FUNCTION_BLOCK "SIKO_DRV_POS_AG04B"
TITLE =
//KNOW_HOW_PROTECT
VERSION : 0.1


VAR_INPUT
  STARTADDRESS_STW : WORD ;	//PERIPHERY_STARTADDRESS_CONTROLBLOCK [HEX ]
  STARTADDRESS_ZSW : WORD ;	//PERIPHERY_STARTADDRESS_STATUSBLOCK [HEX ]
  POS_TARGET_VALUE : DINT ;	//Position Target Value -9999999 to 9999999
  OFF1 : BOOL ;	//STW Bit0 1=TRUE: Operating Condition
  OFF2 : BOOL ;	//STW Bit1 1=TRUE: Operating Condition
  OFF3 : BOOL ;	//STW Bit2  (not implemented)
  OPERATION_ENABLE : BOOL ;	//STW Bit3 1=TRUE: Operation Enable Operating Condition
  STOP : BOOL ;	//STW Bit4 1=TRUE: Operating Condition Positioning
  INTERMEDIATE_STOP : BOOL ;	//STW Bit5 1=TRUE: Operating Condition, 0=Positining interrupted
  AKTIVATE_TRAVEL_JOB : BOOL ;	//STW Bit6 Egde Enables New Travelling Job
  ACKNOWLEDGEMENT : BOOL ;	//STW Bit7 1=TRUE: Acklowledge Fault
  INCHING_1 : BOOL ;	//STW Bit8 1=TRUE: Drives Travels Once by Delta-Inch Target Value
  INCHING_2 : BOOL ;	//STW Bit9 1=TRUE: Drives Travels by a-Inch. Dircetion by Bit 15
  Bit10 : BOOL ;	//STW Bit10 Not Supported
  Bit11 : BOOL ;	//STW Bit11 Not Supported
  Bit12 : BOOL ;	//STW Bit12 Not Supported
  Bit13 : BOOL ;	//STW Bit13 Not Supported
  Bit14 : BOOL ;	//STW Bit14 Not Supported
  NEG_INCHING_2 : BOOL ;	//STW Bit15 1=TRUE: Negative Inching 2 Direction
  START_READ : BOOL ;
  START_WRITE : BOOL ;
  ENABLE_CALIBRATION : BOOL ;
END_VAR
VAR_OUTPUT
  POSITION_ACTUAL_VALUE : DINT ;	//Position Actual Value -9999999 to 9999999
  READY_TO_TURN_ON : BOOL ;	//ZSW Bit0 Supply voltage for motor and electronics unit applied
  READY_TO_TURN : BOOL ;	//ZSW Bit1 Supply voltage for motor and electronics unit applied
  OPERATION_ENABLED : BOOL ;	//ZSW Bit2 1=Positioning operation enabled
  ERROR : BOOL ;	//ZSW Bit3 1=Drive faulty and, therefore, out of operation
  NO_OFF_2 : BOOL ;	//ZSW Bit4 1=No pending OFF 2 command
  NO_OFF_3 : BOOL ;	//ZSW Bit5 Not implemented (statically on '1')
  TURN_ON_DISABLED : BOOL ;	//ZSW Bit6 1=Restart only via “OFF 1” with subsequent “On”
  WARNING : BOOL ;	//ZSW Bit7 1=Drive still in operation, no acknowledgement required
  NO_LAG_ERROR : BOOL ;	//ZSW Bit8 1=No lag error present
  GUIDE_REQUIRED : BOOL ;	//ZSW Bit9 Not supported (statically on ‘1’)
  TARGET_POSITION_REACHED : BOOL ;	//ZSW Bit10 1=Position value is at the end of a travel job in  positioning window
  REFERENCE_POINT_SET : BOOL ;	//ZSW Bit11 Not implemented - absolute system (statically on ‘1’).
  ACK_TARGET_VALUE : BOOL ;	//ZSW Bit12 ‘Edge’ acknowledges that a new positioning job was taken over
  DRIVE_STAND_STILL : BOOL ;	//ZSW Bit13 1=Signals standstill in case of intermediate stop and stop
  LIMIT_VALUE_EXCEEDED : BOOL ;	//ZSW Bit14 1=Position limiting value exceeded in pos. or neg. direction.
  READY_TO_TRAVEL : BOOL ;	//ZSW Bit15 1=AG is ready-to-travel if operation has been enabled
  DI_ES1 : BOOL ;	//Digital Input ES1 at AG04B
  DI_ES2 : BOOL ;	//Digital Input ES1 at AG04B
  DI_DI1 : BOOL ;	//Digital Input ES1 at AG04B
  DI_DI2 : BOOL ;	//Digital Input ES1 at AG04B
  DO_DI_ENABLE : BOOL ;	//Status of Enable at AG04B
  DO_MO_TORQUEDEACTIVATION : BOOL ;	//Status of Torque deactivation at AG04B
  COUNT_READ : INT ;
  COUNT_WRITE : INT ;
  Fault_SFC14 : INT ;
  Fault_SFC15 : INT ;
END_VAR
VAR
  Profibus_Address_r : WORD ;	//Address: 918 dez/ 396 hex Profibus Address r
  Operation_Mode_r : WORD  := W#16#2;	//Address: 930 dez/ 3A2 hex Operation Mode r/w
  Operation_Mode_w : WORD  := W#16#2;	//Address: 930 dez/ 3A2 hex Operation Mode r/w
  Fault_Buffer_r : ARRAY  [0 .. 9 ] OF WORD ;
  Number_of_Faults_r : WORD ;	//Address: 952 dez/ 3B8 hex Number of Faults r
  Hardware_Version_r : WORD ;	//Address: 961 dez/ 3C1 hex Hardware Version r
  Software_Version_r : WORD ;	//Address: 965 dez/ 3C5 hex Software Version r
  Parameter_Transfer_w : WORD ;	//Address: 970 dez/ 3CA hex Parameter Transfer w
  Controller_Parameter_P_r : WORD  := W#16#64;	//Address: 1000 dez/ 3E8 hex Controller Parameter P r/w
  Controller_Parameter_P_w : WORD  := W#16#64;	//Address: 1000 dez/ 3E8 hex Controller Parameter P r/w
  Controller_Parameter_I_r : WORD  := W#16#5;	//Address: 1001 dez/ 3E9 hex Controller Parameter I r/w
  Controller_Parameter_I_w : WORD  := W#16#5;	//Address: 1001 dez/ 3E9 hex Controller Parameter I r/w
  Controller_Parameter_D_r : WORD ;	//Address: 1002 dez/ 3EA hex Controller Parameter D r/w
  Controller_Parameter_D_w : WORD ;	//Address: 1002 dez/ 3EA hex Controller Parameter D r/w
  a_Pos_r : WORD  := W#16#32;	//Address: 1003 dez/ 3EB hex a_Pos r/w
  a_Pos_w : WORD  := W#16#32;	//Address: 1003 dez/ 3EB hex a_Pos r/w
  v_Pos_r : WORD  := W#16#1E;	//Address: 1004 dez/ 3EC hex v_Pos r/w
  v_Pos_w : WORD  := W#16#1E;	//Address: 1004 dez/ 3EC hex v_Pos r/w
  a_Rot_r : WORD  := W#16#32;	//Address: 1005 dez/ 3ED hex a_Rot r/w
  a_Rot_w : WORD  := W#16#32;	//Address: 1005 dez/ 3ED hex a_Rot r/w
  reserved_1_r : WORD ;	//Address: 1006 dez/ 3EE hex reserved 1 r/w
  reserved_1_w : WORD ;	//Address: 1006 dez/ 3EE hex reserved 1 r/w
  a_Inch_r : WORD  := W#16#32;	//Address: 1007 dez/ 3EF hex a_Inch r/w
  a_Inch_w : WORD  := W#16#32;	//Address: 1007 dez/ 3EF hex a_Inch r/w
  v_Inch_r : WORD  := W#16#1E;	//Address: 1008 dez/ 3F0 hex v_Inch r/w
  v_Inch_w : WORD  := W#16#1E;	//Address: 1008 dez/ 3F0 hex v_Inch r/w
  Pos_Window_r : WORD  := W#16#A;	//Address: 1009 dez/ 3F1 hex Pos Window r/w
  Pos_Window_w : WORD  := W#16#A;	//Address: 1009 dez/ 3F1 hex Pos Window r/w
  ue_Numerator_r : WORD  := W#16#1;	//Address: 1010 dez/ 3F2 hex ue_Numerator r/w
  ue_Numerator_w : WORD  := W#16#1;	//Address: 1010 dez/ 3F2 hex ue_Numerator r/w
  ue_Denominator_r : WORD  := W#16#1;	//Address: 1011 dez/ 3F3 hex ue_Denominator r/w
  ue_Denominator_w : WORD  := W#16#1;	//Address: 1011 dez/ 3F3 hex ue_Denominator r/w
  Spindle_Pitch_r : WORD ;	//Address: 1012 dez/ 3F4 hex Spindle Pitch r/w
  Spindle_Pitch_w : WORD ;	//Address: 1012 dez/ 3F4 hex Spindle Pitch r/w
  Sence_of_Rotation_r : WORD ;	//Address: 1013 dez/ 3F5 hex Sence of Rotation r/w
  Sence_of_Rotation_w : WORD ;	//Address: 1013 dez/ 3F5 hex Sence of Rotation r/w
  Pos_Type_r : WORD ;	//Address: 1014 dez/ 3F6 hex Pos Type r/w
  Pos_Type_w : WORD ;	//Address: 1014 dez/ 3F6 hex Pos Type r/w
  reserved_2_r : WORD ;	//Address: 1015 dez/ 3F7 hex resereserved 2
  reserved_2_w : WORD ;	//Address: 1015 dez/ 3F7 hex resereserved 2
  Upper_Limit_r : DWORD  := DW#16#186A0;	//Address: 1016 dez/ 3F8 hex Upper Limit r/w
  Upper_Limit_w : DWORD  := DW#16#186A0;	//Address: 1016 dez/ 3F8 hex Upper Limit r/w
  Lower_Limit_r : DWORD  := DW#16#FFFE7960;	//Address: 1017 dez/ 3F9 hex Lower Limit r/w
  Lower_Limit_w : DWORD  := DW#16#FFFE7960;	//Address: 1017 dez/ 3F9 hex Lower Limit r/w
  Calibration_Value_r : DWORD ;	//Address: 1018 dez/ 3FA hex Calibration Value r/w
  Calibration_Value_w : DWORD ;	//Address: 1018 dez/ 3FA hex Calibration Value r/w
  Delta_Inch_r : DWORD  := DW#16#400;	//Address: 1019 dez/ 3FB hex Delta Inch r/w
  Delta_Inch_w : DWORD  := DW#16#400;	//Address: 1019 dez/ 3FB hex Delta Inch r/w
  System_Status_Word_r : WORD ;	//Address: 1020 dez/ 3FC hex System Status Word r
  StoppMode_Inch2_r : WORD ;	//Address: 1021 dez/ 3FD hex Stopp-Mode Inch2 r/w
  StoppMode_Inch2_w : WORD ;	//Address: 1021 dez/ 3FD hex Stopp-Mode Inch2 r/w
  InPos_Mode_r : WORD ;	//Adresse: 1022 dez/ 3FE hex InPos_Mode r/w
  InPos_Mode_w : WORD ;	//Adresse: 1022 dez/ 3FE hex InPos_Mode r/w
  Loop_length_r : WORD  := W#16#200;	//Adresse: 1023 dez/ 3FF hex Loop_length r/w
  Loop_length_w : WORD  := W#16#200;	//Adresse: 1023 dez/ 3FF hex Loop_length r/w
  Contouring_error_limit_r : WORD  := W#16#190;	//Adresse: 1024 dez/ 400 hex Loop_length r/w
  Contouring_error_limit_w : WORD  := W#16#190;	//Adresse: 1024 dez/ 400 hex Loop_length r/w
  Contouring_error_r : DWORD ;	//Adresse: 1025 dez/ 401 hex Contouring_error r
  Supply_voltage_r : WORD ;	//Adresse: 1026 dez/ 402 hex Supply_voltage r
  Device_temperature_r : WORD ;	//Adresse: 1027 dez/ 403 hex Device_temperature r
  Device_temperature_max_r : WORD ;	//Adresse: 1028 dez/ 404 hex Device_temperature_max r
  Motor_current_r : WORD ;	//Adresse: 1029 dez/ 405 hex Motor_current r
  Motor_current_max_r : WORD ;	//Adresse: 1030 dez/ 406 hex Motor_current_max r
  Gen_Status_Register_r : WORD ;	//Adresse: 1031 dez/ 407 hex Digital_inputs r
  Torque_Deactivation_r : WORD  := W#16#7D;	//Adresse: 1032 dez/ 408 hex InPos_Mode r/w
  Torque_Deactivation_w : WORD  := W#16#7D;	//Adresse: 1032 dez/ 408 hex InPos_Mode r/w
  Serial_number_r : DWORD ;	//Adresse: 1033 dez/ 409 hex Serial_number r
  AF_OSR_START_WRITE : BOOL ;
  OSR_START_WRITE : BOOL ;
  AF_OSR_START_READ : BOOL ;
  OSR_START_READ : BOOL ;
  REFRESH : BOOL ;
  COUNTER_READ : INT ;
  COUNTER_WRITE : INT ;
END_VAR
VAR_TEMP
  DC_STEUERBEREICH_TEMP : ARRAY  [1 .. 14 ] OF //PERIEPHERIE_STEUERBEREICH_TEMP
  BYTE ;
  DC_ZUSTANDSBEREICH_TEMP : ARRAY  [1 .. 14 ] OF //PERIEPHERIE_ZUSTANDSBEREICH_TEMP
  BYTE ;
  Failure : INT ;
END_VAR
BEGIN
NETWORK
TITLE =STW 1
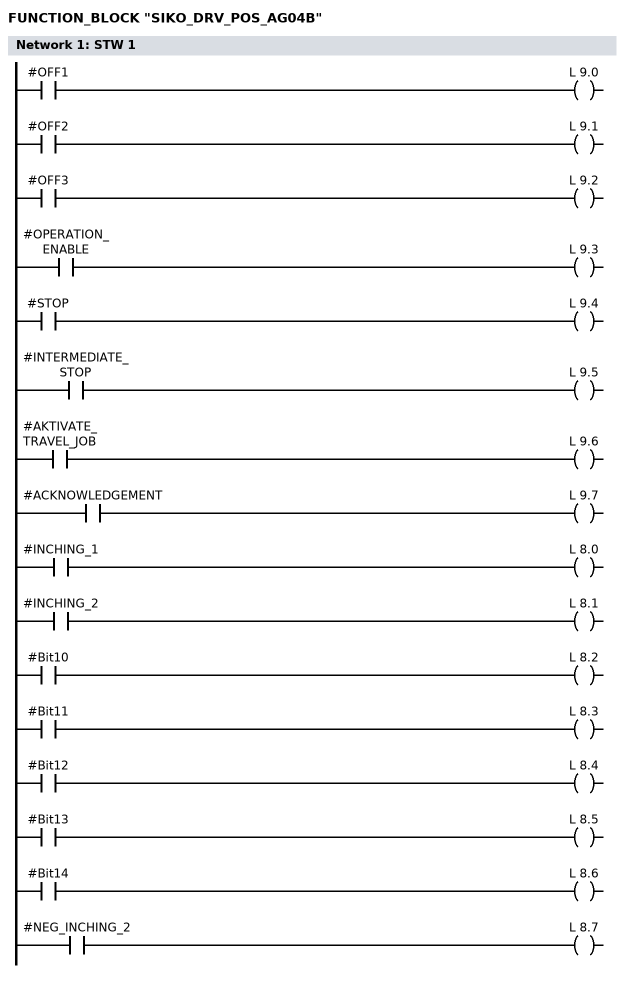
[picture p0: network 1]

      U     #OFF1;
      =     L      9.0;
      U     #OFF2;
      =     L      9.1;
      U     #OFF3;
      =     L      9.2;
      U     #OPERATION_ENABLE;
      =     L      9.3;
      U     #STOP;
      =     L      9.4;
      U     #INTERMEDIATE_STOP;
      =     L      9.5;
      U     #AKTIVATE_TRAVEL_JOB;
      =     L      9.6;
      U     #ACKNOWLEDGEMENT;
      =     L      9.7;
      U     #INCHING_1;
      =     L      8.0;
      U     #INCHING_2;
      =     L      8.1;
      U     #Bit10;
      =     L      8.2;
      U     #Bit11;
      =     L      8.3;
      U     #Bit12;
      =     L      8.4;
      U     #Bit13;
      =     L      8.5;
      U     #Bit14;
      =     L      8.6;
      U     #NEG_INCHING_2;
      =     L      8.7;

NETWORK
TITLE =CREATION OF SET POINT WORD (HSW/PZD2)
//PZD2
      L     #POS_TARGET_VALUE;
      L     L#-9999999;
      >D    ;
      SPB   M001;
      L     0;
      SPA   END0;
M001: L     #POS_TARGET_VALUE;
      L     L#9999999;
      <=D   ;
      SPB   M002;
      L     0;
      SPA   END0;
M002: L     #POS_TARGET_VALUE;
END0: T     LD    10;

NETWORK
TITLE =Start Read / Write Flanke
//Flanke bilden start lesen
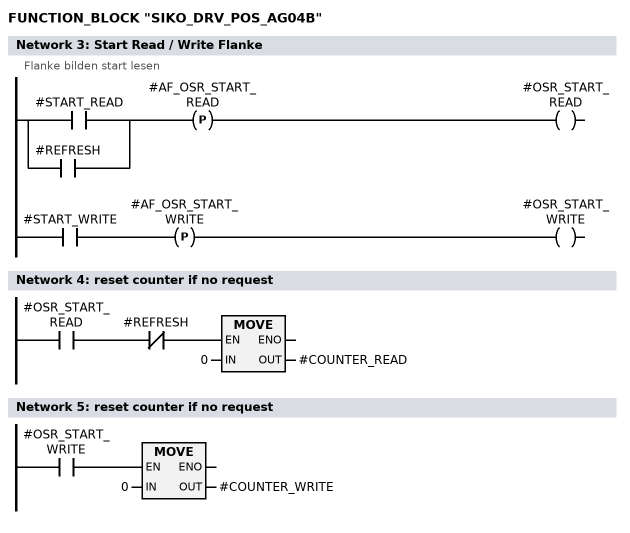
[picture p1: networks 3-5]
      O     #START_READ;
      O     #REFRESH;
      FP    #AF_OSR_START_READ;
      =     #OSR_START_READ;

//Flanke bilden start lesen
      U     #START_WRITE;
      FP    #AF_OSR_START_WRITE;
      =     #OSR_START_WRITE;



NETWORK
TITLE =reset counter if no request

      U     #OSR_START_READ;
      UN    #REFRESH;
      SPBNB _001;
      L     0;
      T     #COUNTER_READ;
_001: NOP   0;
NETWORK
TITLE =reset counter if no request

      U     #OSR_START_WRITE;
      SPBNB _002;
      L     0;
      T     #COUNTER_WRITE;
_002: NOP   0;
NETWORK
TITLE =Par Request read to drv
//
//
//Counter auf 1 bei start
      L     0;
      T     LW     0;
      U     #OSR_START_READ;
      SPBN  pa31;
      L     1;
      T     #COUNTER_READ;



//Parameter anfordern ************************************


//Profibus
pa31: L     #COUNTER_READ;
      L     1;
      ==I   ;
      SPBN  pa32;
      L     W#16#1396;
      T     LW     0;

//Betriebsart
pa32: L     #COUNTER_READ;
      L     2;
      ==I   ;
      SPBN  pa33;
      L     W#16#13A2;
      T     LW     0;

//Störspeicher 0
pa33: L     #COUNTER_READ;
      L     3;
      ==I   ;
      SPBN  pa34;
      L     W#16#63B1;
      T     LW     0;
      L     0;
      T     LW     2;
//Störspeicher 1
pa34: L     #COUNTER_READ;
      L     4;
      ==I   ;
      SPBN  pa35;
      L     W#16#63B1;
      T     LW     0;
      L     1;
      T     LW     2;
//Störspeicher 2
pa35: L     #COUNTER_READ;
      L     5;
      ==I   ;
      SPBN  pa36;
      L     W#16#63B1;
      T     LW     0;
      L     2;
      T     LW     2;
//Störspeicher 3
pa36: L     #COUNTER_READ;
      L     6;
      ==I   ;
      SPBN  pa37;
      L     W#16#63B1;
      T     LW     0;
      L     3;
      T     LW     2;
//Störspeicher 4
pa37: L     #COUNTER_READ;
      L     7;
      ==I   ;
      SPBN  pa38;
      L     W#16#63B1;
      T     LW     0;
      L     4;
      T     LW     2;
//Störspeicher 5
pa38: L     #COUNTER_READ;
      L     8;
      ==I   ;
      SPBN  pa39;
      L     W#16#63B1;
      T     LW     0;
      L     5;
      T     LW     2;
//Störspeicher 6
pa39: L     #COUNTER_READ;
      L     9;
      ==I   ;
      SPBN  pa40;
      L     W#16#63B1;
      T     LW     0;
      L     6;
      T     LW     2;
//Störspeicher 7
pa40: L     #COUNTER_READ;
      L     10;
      ==I   ;
      SPBN  pa41;
      L     W#16#63B1;
      T     LW     0;
      L     7;
      T     LW     2;
//Störspeicher 8
pa41: L     #COUNTER_READ;
      L     11;
      ==I   ;
      SPBN  pa42;
      L     W#16#63B1;
      T     LW     0;
      L     8;
      T     LW     2;
//Störspeicher 9
pa42: L     #COUNTER_READ;
      L     12;
      ==I   ;
      SPBN  pa43;
      L     W#16#63B1;
      T     LW     0;
      L     9;
      T     LW     2;

//Anzahl Störungen
pa43: L     #COUNTER_READ;
      L     13;
      ==I   ;
      SPBN  pa44;
      L     W#16#13B8;
      T     LW     0;

//Hardware-Version
pa44: L     #COUNTER_READ;
      L     14;
      ==I   ;
      SPBN  pa45;
      L     W#16#13C1;
      T     LW     0;

//Software-Version
pa45: L     #COUNTER_READ;
      L     15;
      ==I   ;
      SPBN  pa46;
      L     W#16#13C5;
      T     LW     0;

//Regler-Parameter P-Anteil
pa46: L     #COUNTER_READ;
      L     16;
      ==I   ;
      SPBN  pa47;
      L     W#16#13E8;
      T     LW     0;

//Regler-Parameter I-Anteil
pa47: L     #COUNTER_READ;
      L     17;
      ==I   ;
      SPBN  pa48;
      L     W#16#13E9;
      T     LW     0;

//Regler-Parameter D-Anteil
pa48: L     #COUNTER_READ;
      L     18;
      ==I   ;
      SPBN  pa49;
      L     W#16#13EA;
      T     LW     0;

//a - Pos
pa49: L     #COUNTER_READ;
      L     19;
      ==I   ;
      SPBN  pa50;
      L     W#16#13EB;
      T     LW     0;

//v - Pos
pa50: L     #COUNTER_READ;
      L     20;
      ==I   ;
      SPBN  pa51;
      L     W#16#13EC;
      T     LW     0;

//a - Dreh
pa51: L     #COUNTER_READ;
      L     21;
      ==I   ;
      SPBN  pa52;
      L     W#16#13ED;
      T     LW     0;

//a - Tipp
pa52: L     #COUNTER_READ;
      L     22;
      ==I   ;
      SPBN  pa53;
      L     W#16#13EF;
      T     LW     0;

//v - Tipp
pa53: L     #COUNTER_READ;
      L     23;
      ==I   ;
      SPBN  pa54;
      L     W#16#13F0;
      T     LW     0;

//Pos - Fenster
pa54: L     #COUNTER_READ;
      L     24;
      ==I   ;
      SPBN  pa55;
      L     W#16#13F1;
      T     LW     0;

//ü - Zähler
pa55: L     #COUNTER_READ;
      L     25;
      ==I   ;
      SPBN  pa56;
      L     W#16#13F2;
      T     LW     0;

//ü - Nenner
pa56: L     #COUNTER_READ;
      L     26;
      ==I   ;
      SPBN  pa57;
      L     W#16#13F3;
      T     LW     0;

//Spindelsteigung
pa57: L     #COUNTER_READ;
      L     27;
      ==I   ;
      SPBN  pa58;
      L     W#16#13F4;
      T     LW     0;

//Drehrichtung
pa58: L     #COUNTER_READ;
      L     28;
      ==I   ;
      SPBN  pa59;
      L     W#16#13F5;
      T     LW     0;

//Pos-Art
pa59: L     #COUNTER_READ;
      L     29;
      ==I   ;
      SPBN  pa60;
      L     W#16#13F6;
      T     LW     0;

//Oberer Grenzwert
pa60: L     #COUNTER_READ;
      L     30;
      ==I   ;
      SPBN  pa61;
      L     W#16#13F8;
      T     LW     0;

//Unterer Grenzwert
pa61: L     #COUNTER_READ;
      L     31;
      ==I   ;
      SPBN  pa62;
      L     W#16#13F9;
      T     LW     0;

//Kalibrierwert
pa62: L     #COUNTER_READ;
      L     32;
      ==I   ;
      SPBN  pa63;
      L     W#16#13FA;
      T     LW     0;

//Delta Tipp
pa63: L     #COUNTER_READ;
      L     33;
      ==I   ;
      SPBN  pa64;
      L     W#16#13FB;
      T     LW     0;

//SYSTEM Statuswort
pa64: L     #COUNTER_READ;
      L     34;
      ==I   ;
      SPBN  pa65;
      L     W#16#13FC;
      T     LW     0;

//Stopp-Mode Tipp2
pa65: L     #COUNTER_READ;
      L     35;
      ==I   ;
      SPBN  pa66;
      L     W#16#13FD;
      T     LW     0;

//InPos-Mode
pa66: L     #COUNTER_READ;
      L     36;
      ==I   ;
      SPBN  pa67;
      L     W#16#13FE;
      T     LW     0;

//Schleifenlaenge
pa67: L     #COUNTER_READ;
      L     37;
      ==I   ;
      SPBN  pa68;
      L     W#16#13FF;
      T     LW     0;

//Schleppfehler_Grenze
pa68: L     #COUNTER_READ;
      L     38;
      ==I   ;
      SPBN  pa69;
      L     W#16#1400;
      T     LW     0;

//Schleppfehler
pa69: L     #COUNTER_READ;
      L     39;
      ==I   ;
      SPBN  pa70;
      L     W#16#1401;
      T     LW     0;

//Versorgungsspannung
pa70: L     #COUNTER_READ;
      L     40;
      ==I   ;
      SPBN  pa71;
      L     W#16#1402;
      T     LW     0;

//Geraetetemperatur
pa71: L     #COUNTER_READ;
      L     41;
      ==I   ;
      SPBN  pa72;
      L     W#16#1403;
      T     LW     0;

//Geraetetemperatur_Max
pa72: L     #COUNTER_READ;
      L     42;
      ==I   ;
      SPBN  pa73;
      L     W#16#1404;
      T     LW     0;

//Motorstrom
pa73: L     #COUNTER_READ;
      L     43;
      ==I   ;
      SPBN  pa74;
      L     W#16#1405;
      T     LW     0;

//Motorstrom_Max
pa74: L     #COUNTER_READ;
      L     44;
      ==I   ;
      SPBN  pa75;
      L     W#16#1406;
      T     LW     0;

//Digital_Eingaenge
pa75: L     #COUNTER_READ;
      L     45;
      ==I   ;
      SPBN  pa76;
      L     W#16#1407;
      T     LW     0;

//Drehmoment_Abschaltung
pa76: L     #COUNTER_READ;
      L     46;
      ==I   ;
      SPBN  pa77;
      L     W#16#1408;
      T     LW     0;

//Seriennummer
pa77: L     #COUNTER_READ;
      L     47;
      ==I   ;
      SPBN  pa99;
      L     W#16#1409;
      T     LW     0;

pa99: NOP   0; //ENDE


NETWORK
TITLE =Par Request write to drv
//
//
//
//
//Counter auf 1 bei start
      U     #OSR_START_WRITE;
      SPBN  pr61;
      L     1;
      T     #COUNTER_WRITE;


//Parameter anfordern ************************************
//Betriebsart
pr61: L     #COUNTER_WRITE;
      L     1;
      ==I   ;
      SPBN  pr62;
      L     #Operation_Mode_w;
      L     #Operation_Mode_r;
      ==I   ;
      SPB   co80;
      L     W#16#23A2;
      T     LW     0;
      L     #Operation_Mode_w;
      T     LD     4;

//Reglerparameter_P
pr62: L     #COUNTER_WRITE;
      L     2;
      ==I   ;
      SPBN  pr63;
      L     #Controller_Parameter_P_w;
      L     #Controller_Parameter_P_r;
      ==I   ;
      SPB   co80;
      L     W#16#23E8;
      T     LW     0;
      L     #Controller_Parameter_P_w;
      T     LD     4;

//Reglerparameter_I
pr63: L     #COUNTER_WRITE;
      L     3;
      ==I   ;
      SPBN  pr64;
      L     #Controller_Parameter_I_w;
      L     #Controller_Parameter_I_r;
      ==I   ;
      SPB   co80;
      L     W#16#23E9;
      T     LW     0;
      L     #Controller_Parameter_I_w;
      T     LD     4;

//Reglerparameter_D
pr64: L     #COUNTER_WRITE;
      L     4;
      ==I   ;
      SPBN  pr65;
      L     #Controller_Parameter_D_w;
      L     #Controller_Parameter_D_r;
      ==I   ;
      SPB   co80;
      L     W#16#23EA;
      T     LW     0;
      L     #Controller_Parameter_D_w;
      T     LD     4;

//a_Pos
pr65: L     #COUNTER_WRITE;
      L     5;
      ==I   ;
      SPBN  pr66;
      L     #a_Pos_w;
      L     #a_Pos_r;
      ==I   ;
      SPB   co80;
      L     W#16#23EB;
      T     LW     0;
      L     #a_Pos_w;
      T     LD     4;

//v_Pos
pr66: L     #COUNTER_WRITE;
      L     6;
      ==I   ;
      SPBN  pr67;
      L     #v_Pos_w;
      L     #v_Pos_r;
      ==I   ;
      SPB   co80;
      L     W#16#23EC;
      T     LW     0;
      L     #v_Pos_w;
      T     LD     4;

//a_Dreh
pr67: L     #COUNTER_WRITE;
      L     7;
      ==I   ;
      SPBN  pr68;
      L     #a_Rot_w;
      L     #a_Rot_r;
      ==I   ;
      SPB   co80;
      L     W#16#23ED;
      T     LW     0;
      L     #a_Rot_w;
      T     LD     4;

//a_Tipp
pr68: L     #COUNTER_WRITE;
      L     8;
      ==I   ;
      SPBN  pr69;
      L     #a_Inch_w;
      L     #a_Inch_r;
      ==I   ;
      SPB   co80;
      L     W#16#23EF;
      T     LW     0;
      L     #a_Inch_w;
      T     LD     4;

//v_Tip
pr69: L     #COUNTER_WRITE;
      L     9;
      ==I   ;
      SPBN  pr70;
      L     #v_Inch_w;
      L     #v_Inch_r;
      ==I   ;
      SPB   co80;
      L     W#16#23F0;
      T     LW     0;
      L     #v_Inch_w;
      T     LD     4;

//Pos_Fenster
pr70: L     #COUNTER_WRITE;
      L     10;
      ==I   ;
      SPBN  pr71;
      L     #Pos_Window_w;
      L     #Pos_Window_r;
      ==I   ;
      SPB   co80;
      L     W#16#23F1;
      T     LW     0;
      L     #Pos_Window_w;
      T     LD     4;

//ue_Zaehler
pr71: L     #COUNTER_WRITE;
      L     11;
      ==I   ;
      SPBN  pr72;
      L     #ue_Numerator_w;
      L     #ue_Numerator_r;
      ==I   ;
      SPB   co80;
      L     W#16#23F2;
      T     LW     0;
      L     #ue_Numerator_w;
      T     LD     4;

//ue_Nenner
pr72: L     #COUNTER_WRITE;
      L     12;
      ==I   ;
      SPBN  pr73;
      L     #ue_Denominator_w;
      L     #ue_Denominator_r;
      ==I   ;
      SPB   co80;
      L     W#16#23F3;
      T     LW     0;
      L     #ue_Denominator_w;
      T     LD     4;

//Spindelsteigung
pr73: L     #COUNTER_WRITE;
      L     13;
      ==I   ;
      SPBN  pr74;
      L     #Spindle_Pitch_w;
      L     #Spindle_Pitch_r;
      ==I   ;
      SPB   co80;
      L     W#16#23F4;
      T     LW     0;
      L     #Spindle_Pitch_w;
      T     LD     4;

//Drehrichtung
pr74: L     #COUNTER_WRITE;
      L     14;
      ==I   ;
      SPBN  pr75;
      L     #Sence_of_Rotation_w;
      L     #Sence_of_Rotation_r;
      ==I   ;
      SPB   co80;
      L     W#16#23F5;
      T     LW     0;
      L     #Sence_of_Rotation_w;
      T     LD     4;

//Pos_Art_
pr75: L     #COUNTER_WRITE;
      L     15;
      ==I   ;
      SPBN  pr76;
      L     #Pos_Type_w;
      L     #Pos_Type_r;
      ==I   ;
      SPB   co80;
      L     W#16#23F6;
      T     LW     0;
      L     #Pos_Type_w;
      T     LD     4;

//oberer_Grenzwert
pr76: L     #COUNTER_WRITE;
      L     16;
      ==I   ;
      SPBN  pr77;
      L     #Upper_Limit_w;
      L     #Upper_Limit_r;
      ==I   ;
      SPB   co80;
      L     W#16#33F8;
      T     LW     0;
      L     #Upper_Limit_w;
      T     LD     4;

//unterer_Grenzwert
pr77: L     #COUNTER_WRITE;
      L     17;
      ==I   ;
      SPBN  pr78;
      L     #Lower_Limit_w;
      L     #Lower_Limit_r;
      ==I   ;
      SPB   co80;
      L     W#16#33F9;
      T     LW     0;
      L     #Lower_Limit_w;
      T     LD     4;

//Kalibrierwert
pr78: L     #COUNTER_WRITE;
      L     18;
      ==I   ;
      SPBN  pr79;
//L     #Calibration_Value_w
//L     #Calibration_Value_r
//==I
      UN    #ENABLE_CALIBRATION;
      SPB   co80;
      L     W#16#33FA;
      T     LW     0;
      L     #Calibration_Value_w;
      T     LD     4;

//Delta_Tipp
pr79: L     #COUNTER_WRITE;
      L     19;
      ==I   ;
      SPBN  pr80;
      L     #Delta_Inch_w;
      L     #Delta_Inch_r;
      ==I   ;
      SPB   co80;
      L     W#16#33FB;
      T     LW     0;
      L     #Delta_Inch_w;
      T     LD     4;

//Stopp-Mode Tipp2
pr80: L     #COUNTER_WRITE;
      L     20;
      ==I   ;
      SPBN  pr81;
      L     #StoppMode_Inch2_w;
      L     #StoppMode_Inch2_r;
      ==I   ;
      SPB   co80;
      L     W#16#23FD;
      T     LW     0;
      L     #StoppMode_Inch2_w;
      T     LD     4;

//InPos_Mode
pr81: L     #COUNTER_WRITE;
      L     21;
      ==I   ;
      SPBN  pl82;
      L     #InPos_Mode_w;
      L     #InPos_Mode_r;
      ==I   ;
      SPB   co80;
      L     W#16#23FE;
      T     LW     0;
      L     #InPos_Mode_w;
      T     LD     4;

//Schleifenlaenge
pl82: L     #COUNTER_WRITE;
      L     22;
      ==I   ;
      SPBN  pl83;
      L     #Loop_length_w;
      L     #Loop_length_r;
      ==I   ;
      SPB   co80;
      L     W#16#23FF;
      T     LW     0;
      L     #Loop_length_w;
      T     LD     4;

//Schleppfehler_Grenze
pl83: L     #COUNTER_WRITE;
      L     23;
      ==I   ;
      SPBN  pl84;
      L     #Contouring_error_limit_w;
      L     #Contouring_error_limit_r;
      ==I   ;
      SPB   co80;
      L     W#16#2400;
      T     LW     0;
      L     #Contouring_error_limit_w;
      T     LD     4;

//Drehmoment_Abschaltung
pl84: L     #COUNTER_WRITE;
      L     24;
      ==I   ;
      SPBN  pz99;
      L     #Torque_Deactivation_w;
      L     #Torque_Deactivation_r;
      ==I   ;
      SPB   co80;
      L     W#16#2408;
      T     LW     0;
      L     #Torque_Deactivation_w;
      T     LD     4;

//Parametersatz laden
pz99: L     #COUNTER_WRITE;
      L     25;
      ==I   ;
      SPBN  end6;
      L     W#16#23CA;
      T     LW     0;
      L     #Parameter_Transfer_w;
      T     LD     4;

      SPA   end6;


//erhöhe Zähler wenn kein schreiben notwendig
// Zähler +1
co80: L     #COUNTER_WRITE;
      INC   1;
      T     #COUNTER_WRITE;

end6: NOP   0; //ENDE



NETWORK
TITLE =
//Eingänge abfragen, wenn Parameterabgleich inaktiv
      L     0;
      L     #COUNT_WRITE;
      ==I   ;
      SPBN  xyy1;
      L     0;
      L     #COUNT_READ;
      ==I   ;
      SPBN  xyy1;
      L     W#16#1407;
      T     LW     0;

xyy1: NOP   0;


NETWORK
TITLE =transmit to drive

      CALL "DPWR_DAT" (
           LADDR                    := #STARTADDRESS_STW,
           RECORD                   := P#L 0.0 BYTE 14,
           RET_VAL                  := #Fault_SFC15);
      NOP   0;
NETWORK
TITLE =Read from Drive

      CALL "DPRD_DAT" (
           LADDR                    := #STARTADDRESS_ZSW,
           RET_VAL                  := #Fault_SFC14,
           RECORD                   := P#L 14.0 BYTE 14);
      NOP   0;

NETWORK
TITLE =
//Eingänge abfragen, wenn Parameterabgleich inaktiv
      L     0;
      L     #COUNT_WRITE;
      ==I   ;
      SPBN  xxy1;
      L     0;
      L     #COUNT_READ;
      ==I   ;
      SPBN  xxy1;
      L     LW    14;
      L     W#16#1407;
      ==I   ;
      SPBN  xxy1;

      U     L     21.0;
      =     #DI_ES1;
      U     L     21.1;
      =     #DI_ES2;
      U     L     21.2;
      =     #DI_DI1;
      U     L     21.3;
      =     #DI_DI2;
      U     L     21.4;
      =     #DO_DI_ENABLE;
      U     L     21.7;
      =     #DO_MO_TORQUEDEACTIVATION;

xxy1: NOP   0;


NETWORK
TITLE =read par from drv (read)
//
//
      L     #COUNTER_READ; //Zählerstand nach aussen geben
      T     #COUNT_READ; //Zählerstand nach aussen geben
//Profibus
      L     #COUNTER_READ; //Parameterwert auslesen START
      L     1;
      ==I   ;
      SPBN  rp2;
      L     LW    14;
      L     W#16#1396;
      ==I   ;
      SPBN  end9;
      L     LD    18;
      T     #Profibus_Address_r;
// Zähler +1
      L     #COUNTER_READ;
      INC   1;
      T     #COUNTER_READ; //Parameterwert auslesen ENDE

//Betriebsart
rp2:  L     #COUNTER_READ; //Parameterwert auslesen START
      L     2;
      ==I   ;
      SPBN  rp3;
      L     LW    14;
      L     W#16#13A2;
      ==I   ;
      SPBN  end9;
      L     LD    18;
      T     #Operation_Mode_r;
// Zähler +1
      L     #COUNTER_READ;
      INC   1;
      T     #COUNTER_READ; //Parameterwert auslesen ENDE

//Störspeicher 0
rp3:  L     #COUNTER_READ; //Parameterwert auslesen START
      L     3;
      ==I   ;
      SPBN  rp4;
      L     LW    14;
      L     W#16#43B1;
      ==I   ;
      SPBN  end9;
      L     LW    16;
      L     0;
      ==I   ;
      SPBN  end9;
      L     LD    18;
      T     #Fault_Buffer_r[0];
// Zähler +1
      L     #COUNTER_READ;
      INC   1;
      T     #COUNTER_READ; //Parameterwert auslesen ENDE

//Störspeicher 1
rp4:  L     #COUNTER_READ; //Parameterwert auslesen START
      L     4;
      ==I   ;
      SPBN  rp5;
      L     LW    14;
      L     W#16#43B1;
      ==I   ;
      SPBN  end9;
      L     LW    16;
      L     1;
      ==I   ;
      SPBN  end9;
      L     LD    18;
      T     #Fault_Buffer_r[1];
// Zähler +1
      L     #COUNTER_READ;
      INC   1;
      T     #COUNTER_READ; //Parameterwert auslesen ENDE

//Störspeicher 2
rp5:  L     #COUNTER_READ; //Parameterwert auslesen START
      L     5;
      ==I   ;
      SPBN  rp6;
      L     LW    14;
      L     W#16#43B1;
      ==I   ;
      SPBN  end9;
      L     LW    16;
      L     2;
      ==I   ;
      SPBN  end9;
      L     LD    18;
      T     #Fault_Buffer_r[2];
// Zähler +1
      L     #COUNTER_READ;
      INC   1;
      T     #COUNTER_READ; //Parameterwert auslesen ENDE

//Störspeicher 3
rp6:  L     #COUNTER_READ; //Parameterwert auslesen START
      L     6;
      ==I   ;
      SPBN  rp7;
      L     LW    14;
      L     W#16#43B1;
      ==I   ;
      SPBN  end9;
      L     LW    16;
      L     3;
      ==I   ;
      SPBN  end9;
      L     LD    18;
      T     #Fault_Buffer_r[3];
// Zähler +1
      L     #COUNTER_READ;
      INC   1;
      T     #COUNTER_READ; //Parameterwert auslesen ENDE

//Störspeicher 4
rp7:  L     #COUNTER_READ; //Parameterwert auslesen START
      L     7;
      ==I   ;
      SPBN  rp8;
      L     LW    14;
      L     W#16#43B1;
      ==I   ;
      SPBN  end9;
      L     LW    16;
      L     4;
      ==I   ;
      SPBN  end9;
      L     LD    18;
      T     #Fault_Buffer_r[4];
// Zähler +1
      L     #COUNTER_READ;
      INC   1;
      T     #COUNTER_READ; //Parameterwert auslesen ENDE

//Störspeicher 5
rp8:  L     #COUNTER_READ; //Parameterwert auslesen START
      L     8;
      ==I   ;
      SPBN  rp9;
      L     LW    14;
      L     W#16#43B1;
      ==I   ;
      SPBN  end9;
      L     LW    16;
      L     5;
      ==I   ;
      SPBN  end9;
      L     LD    18;
      T     #Fault_Buffer_r[5];
// Zähler +1
      L     #COUNTER_READ;
      INC   1;
      T     #COUNTER_READ; //Parameterwert auslesen ENDE

//Störspeicher 6
rp9:  L     #COUNTER_READ; //Parameterwert auslesen START
      L     9;
      ==I   ;
      SPBN  rp10;
      L     LW    14;
      L     W#16#43B1;
      ==I   ;
      SPBN  end9;
      L     LW    16;
      L     6;
      ==I   ;
      SPBN  end9;
      L     LD    18;
      T     #Fault_Buffer_r[6];
// Zähler +1
      L     #COUNTER_READ;
      INC   1;
      T     #COUNTER_READ; //Parameterwert auslesen ENDE

//Störspeicher 7
rp10: L     #COUNTER_READ; //Parameterwert auslesen START
      L     10;
      ==I   ;
      SPBN  rp11;
      L     LW    14;
      L     W#16#43B1;
      ==I   ;
      SPBN  end9;
      L     LW    16;
      L     7;
      ==I   ;
      SPBN  end9;
      L     LD    18;
      T     #Fault_Buffer_r[7];
// Zähler +1
      L     #COUNTER_READ;
      INC   1;
      T     #COUNTER_READ; //Parameterwert auslesen ENDE

//Störspeicher 8
rp11: L     #COUNTER_READ; //Parameterwert auslesen START
      L     11;
      ==I   ;
      SPBN  rp12;
      L     LW    14;
      L     W#16#43B1;
      ==I   ;
      SPBN  end9;
      L     LW    16;
      L     8;
      ==I   ;
      SPBN  end9;
      L     LD    18;
      T     #Fault_Buffer_r[8];
// Zähler +1
      L     #COUNTER_READ;
      INC   1;
      T     #COUNTER_READ; //Parameterwert auslesen ENDE

//Störspeicher 9
rp12: L     #COUNTER_READ; //Parameterwert auslesen START
      L     12;
      ==I   ;
      SPBN  rp13;
      L     LW    14;
      L     W#16#43B1;
      ==I   ;
      SPBN  end9;
      L     LW    16;
      L     9;
      ==I   ;
      SPBN  end9;
      L     LD    18;
      T     #Fault_Buffer_r[9];
// Zähler +1
      L     #COUNTER_READ;
      INC   1;
      T     #COUNTER_READ; //Parameterwert auslesen ENDE

//Anzahl Störungen
rp13: L     #COUNTER_READ; //Parameterwert auslesen START
      L     13;
      ==I   ;
      SPBN  rp14;
      L     LW    14;
      L     W#16#13B8;
      ==I   ;
      SPBN  end9;
      L     LD    18;
      T     #Number_of_Faults_r;
// Zähler +1
      L     #COUNTER_READ;
      INC   1;
      T     #COUNTER_READ; //Parameterwert auslesen ENDE

//Hardware-Version
rp14: L     #COUNTER_READ; //Parameterwert auslesen START
      L     14;
      ==I   ;
      SPBN  rp15;
      L     LW    14;
      L     W#16#13C1;
      ==I   ;
      SPBN  end9;
      L     LD    18;
      T     #Hardware_Version_r;
// Zähler +1
      L     #COUNTER_READ;
      INC   1;
      T     #COUNTER_READ; //Parameterwert auslesen ENDE

//Software-Version
rp15: L     #COUNTER_READ; //Parameterwert auslesen START
      L     15;
      ==I   ;
      SPBN  rp16;
      L     LW    14;
      L     W#16#13C5;
      ==I   ;
      SPBN  end9;
      L     LD    18;
      T     #Software_Version_r;
// Zähler +1
      L     #COUNTER_READ;
      INC   1;
      T     #COUNTER_READ; //Parameterwert auslesen ENDE

//Regler-Parameter P-Anteil
rp16: L     #COUNTER_READ; //Parameterwert auslesen START
      L     16;
      ==I   ;
      SPBN  rp17;
      L     LW    14;
      L     W#16#13E8;
      ==I   ;
      SPBN  end9;
      L     LD    18;
      T     #Controller_Parameter_P_r;
// Zähler +1
      L     #COUNTER_READ;
      INC   1;
      T     #COUNTER_READ; //Parameterwert auslesen ENDE

//Regler-Parameter I-Anteil
rp17: L     #COUNTER_READ; //Parameterwert auslesen START
      L     17;
      ==I   ;
      SPBN  rp18;
      L     LW    14;
      L     W#16#13E9;
      ==I   ;
      SPBN  end9;
      L     LD    18;
      T     #Controller_Parameter_I_r;
// Zähler +1
      L     #COUNTER_READ;
      INC   1;
      T     #COUNTER_READ; //Parameterwert auslesen ENDE

//Regler-Parameter D-Anteil
rp18: L     #COUNTER_READ; //Parameterwert auslesen START
      L     18;
      ==I   ;
      SPBN  rp19;
      L     LW    14;
      L     W#16#13EA;
      ==I   ;
      SPBN  end9;
      L     LD    18;
      T     #Controller_Parameter_D_r;
// Zähler +1
      L     #COUNTER_READ;
      INC   1;
      T     #COUNTER_READ; //Parameterwert auslesen ENDE

//a - Pos
rp19: L     #COUNTER_READ; //Parameterwert auslesen START
      L     19;
      ==I   ;
      SPBN  rp20;
      L     LW    14;
      L     W#16#13EB;
      ==I   ;
      SPBN  end9;
      L     LD    18;
      T     #a_Pos_r;
// Zähler +1
      L     #COUNTER_READ;
      INC   1;
      T     #COUNTER_READ; //Parameterwert auslesen ENDE

//v - Pos
rp20: L     #COUNTER_READ; //Parameterwert auslesen START
      L     20;
      ==I   ;
      SPBN  rp21;
      L     LW    14;
      L     W#16#13EC;
      ==I   ;
      SPBN  end9;
      L     LD    18;
      T     #v_Pos_r;
// Zähler +1
      L     #COUNTER_READ;
      INC   1;
      T     #COUNTER_READ; //Parameterwert auslesen ENDE

//a - Dreh
rp21: L     #COUNTER_READ; //Parameterwert auslesen START
      L     21;
      ==I   ;
      SPBN  rp22;
      L     LW    14;
      L     W#16#13ED;
      ==I   ;
      SPBN  end9;
      L     LD    18;
      T     #a_Rot_r;
// Zähler +1
      L     #COUNTER_READ;
      INC   1;
      T     #COUNTER_READ; //Parameterwert auslesen ENDE

//a - Tipp
rp22: L     #COUNTER_READ; //Parameterwert auslesen START
      L     22;
      ==I   ;
      SPBN  rp23;
      L     LW    14;
      L     W#16#13EF;
      ==I   ;
      SPBN  end9;
      L     LD    18;
      T     #a_Inch_r;
// Zähler +1
      L     #COUNTER_READ;
      INC   1;
      T     #COUNTER_READ; //Parameterwert auslesen ENDE

//v - Tipp
rp23: L     #COUNTER_READ; //Parameterwert auslesen START
      L     23;
      ==I   ;
      SPBN  rp24;
      L     LW    14;
      L     W#16#13F0;
      ==I   ;
      SPBN  end9;
      L     LD    18;
      T     #v_Inch_r;
// Zähler +1
      L     #COUNTER_READ;
      INC   1;
      T     #COUNTER_READ; //Parameterwert auslesen ENDE

//Pos - Fenster
rp24: L     #COUNTER_READ; //Parameterwert auslesen START
      L     24;
      ==I   ;
      SPBN  rp25;
      L     LW    14;
      L     W#16#13F1;
      ==I   ;
      SPBN  end9;
      L     LD    18;
      T     #Pos_Window_r;
// Zähler +1
      L     #COUNTER_READ;
      INC   1;
      T     #COUNTER_READ; //Parameterwert auslesen ENDE

//ü - Zähler
rp25: L     #COUNTER_READ; //Parameterwert auslesen START
      L     25;
      ==I   ;
      SPBN  rp26;
      L     LW    14;
      L     W#16#13F2;
      ==I   ;
      SPBN  end9;
      L     LD    18;
      T     #ue_Numerator_r;
// Zähler +1
      L     #COUNTER_READ;
      INC   1;
      T     #COUNTER_READ; //Parameterwert auslesen ENDE

//ü - Nenner
rp26: L     #COUNTER_READ; //Parameterwert auslesen START
      L     26;
      ==I   ;
      SPBN  rp27;
      L     LW    14;
      L     W#16#13F3;
      ==I   ;
      SPBN  end9;
      L     LD    18;
      T     #ue_Denominator_r;
// Zähler +1
      L     #COUNTER_READ;
      INC   1;
      T     #COUNTER_READ; //Parameterwert auslesen ENDE

//Spindelsteigung
rp27: L     #COUNTER_READ; //Parameterwert auslesen START
      L     27;
      ==I   ;
      SPBN  rp28;
      L     LW    14;
      L     W#16#13F4;
      ==I   ;
      SPBN  end9;
      L     LD    18;
      T     #Spindle_Pitch_r;
// Zähler +1
      L     #COUNTER_READ;
      INC   1;
      T     #COUNTER_READ; //Parameterwert auslesen ENDE

//Drehrichtung
rp28: L     #COUNTER_READ; //Parameterwert auslesen START
      L     28;
      ==I   ;
      SPBN  rp29;
      L     LW    14;
      L     W#16#13F5;
      ==I   ;
      SPBN  end9;
      L     LD    18;
      T     #Sence_of_Rotation_r;
// Zähler +1
      L     #COUNTER_READ;
      INC   1;
      T     #COUNTER_READ; //Parameterwert auslesen ENDE

//Pos-Art
rp29: L     #COUNTER_READ; //Parameterwert auslesen START
      L     29;
      ==I   ;
      SPBN  rp30;
      L     LW    14;
      L     W#16#13F6;
      ==I   ;
      SPBN  end9;
      L     LD    18;
      T     #Pos_Type_r;
// Zähler +1
      L     #COUNTER_READ;
      INC   1;
      T     #COUNTER_READ; //Parameterwert auslesen ENDE

//Oberer Grenzwert
rp30: L     #COUNTER_READ; //Parameterwert auslesen START
      L     30;
      ==I   ;
      SPBN  rp31;
      L     LW    14;
      L     W#16#23F8;
      ==I   ;
      SPBN  end9;
      L     LD    18;
      T     #Upper_Limit_r;
// Zähler +1
      L     #COUNTER_READ;
      INC   1;
      T     #COUNTER_READ; //Parameterwert auslesen ENDE

//Unterer Grenzwert
rp31: L     #COUNTER_READ; //Parameterwert auslesen START
      L     31;
      ==I   ;
      SPBN  rp32;
      L     LW    14;
      L     W#16#23F9;
      ==I   ;
      SPBN  end9;
      L     LD    18;
      T     #Lower_Limit_r;
// Zähler +1
      L     #COUNTER_READ;
      INC   1;
      T     #COUNTER_READ; //Parameterwert auslesen ENDE

//Kalibrierwert
rp32: L     #COUNTER_READ; //Parameterwert auslesen START
      L     32;
      ==I   ;
      SPBN  rp33;
      L     LW    14;
      L     W#16#23FA;
      ==I   ;
      SPBN  end9;
      L     LD    18;
      T     #Calibration_Value_r;
// Zähler +1
      L     #COUNTER_READ;
      INC   1;
      T     #COUNTER_READ; //Parameterwert auslesen ENDE

//Delta Tipp
rp33: L     #COUNTER_READ; //Parameterwert auslesen START
      L     33;
      ==I   ;
      SPBN  rp34;
      L     LW    14;
      L     W#16#23FB;
      ==I   ;
      SPBN  end9;
      L     LD    18;
      T     #Delta_Inch_r;
// Zähler +1
      L     #COUNTER_READ;
      INC   1;
      T     #COUNTER_READ; //Parameterwert auslesen ENDE

//SYSTEM Statuswort
rp34: L     #COUNTER_READ; //Parameterwert auslesen START
      L     34;
      ==I   ;
      SPBN  rp35;
      L     LW    14;
      L     W#16#13FC;
      ==I   ;
      SPBN  end9;
      L     LD    18;
      T     #System_Status_Word_r;
// Zähler +1
      L     #COUNTER_READ;
      INC   1;
      T     #COUNTER_READ; //Parameterwert auslesen ENDE

//Stopp-Mode Tipp2
rp35: L     #COUNTER_READ; //Parameterwert auslesen START
      L     35;
      ==I   ;
      SPBN  rp36;
      L     LW    14;
      L     W#16#13FD;
      ==I   ;
      SPBN  end9;
      L     LD    18;
      T     #StoppMode_Inch2_r;
// Zähler +1
      L     #COUNTER_READ;
      INC   1;
      T     #COUNTER_READ; //Parameterwert auslesen ENDE

//InPos_Mode
rp36: L     #COUNTER_READ; //Parameterwert auslesen START
      L     36;
      ==I   ;
      SPBN  rp37;
      L     LW    14;
      L     W#16#13FE;
      ==I   ;
      SPBN  end9;
      L     LD    18;
      T     #InPos_Mode_r;
// Zähler +1
      L     #COUNTER_READ;
      INC   1;
      T     #COUNTER_READ; //Parameterwert auslesen ENDE

//Schleifenlaenge
rp37: L     #COUNTER_READ; //Parameterwert auslesen START
      L     37;
      ==I   ;
      SPBN  rp38;
      L     LW    14;
      L     W#16#13FF;
      ==I   ;
      SPBN  end9;
      L     LD    18;
      T     #Loop_length_r;
// Zähler +1
      L     #COUNTER_READ;
      INC   1;
      T     #COUNTER_READ; //Parameterwert auslesen ENDE

//Schleppfehler_Grenze
rp38: L     #COUNTER_READ; //Parameterwert auslesen START
      L     38;
      ==I   ;
      SPBN  rp39;
      L     LW    14;
      L     W#16#1400;
      ==I   ;
      SPBN  end9;
      L     LD    18;
      T     #Contouring_error_limit_r;
// Zähler +1
      L     #COUNTER_READ;
      INC   1;
      T     #COUNTER_READ; //Parameterwert auslesen ENDE

//Schleppfehler DWORD
rp39: L     #COUNTER_READ; //Parameterwert auslesen START
      L     39;
      ==I   ;
      SPBN  rp40;
      L     LW    14;
      L     W#16#2401;
      ==I   ;
      SPBN  end9;
      L     LD    18;
      T     #Contouring_error_r;
// Zähler +1
      L     #COUNTER_READ;
      INC   1;
      T     #COUNTER_READ; //Parameterwert auslesen ENDE

//Versorgungsspannung
rp40: L     #COUNTER_READ; //Parameterwert auslesen START
      L     40;
      ==I   ;
      SPBN  rp41;
      L     LW    14;
      L     W#16#1402;
      ==I   ;
      SPBN  end9;
      L     LD    18;
      T     #Supply_voltage_r;
// Zähler +1
      L     #COUNTER_READ;
      INC   1;
      T     #COUNTER_READ; //Parameterwert auslesen ENDE

//Geraetetemperatur
rp41: L     #COUNTER_READ; //Parameterwert auslesen START
      L     41;
      ==I   ;
      SPBN  rp42;
      L     LW    14;
      L     W#16#1403;
      ==I   ;
      SPBN  end9;
      L     LD    18;
      T     #Device_temperature_r;
// Zähler +1
      L     #COUNTER_READ;
      INC   1;
      T     #COUNTER_READ; //Parameterwert auslesen ENDE

//Geraetetemperatur_Max
rp42: L     #COUNTER_READ; //Parameterwert auslesen START
      L     42;
      ==I   ;
      SPBN  rp43;
      L     LW    14;
      L     W#16#1404;
      ==I   ;
      SPBN  end9;
      L     LD    18;
      T     #Device_temperature_max_r;
// Zähler +1
      L     #COUNTER_READ;
      INC   1;
      T     #COUNTER_READ; //Parameterwert auslesen ENDE

//Motorstrom
rp43: L     #COUNTER_READ; //Parameterwert auslesen START
      L     43;
      ==I   ;
      SPBN  rp44;
      L     LW    14;
      L     W#16#1405;
      ==I   ;
      SPBN  end9;
      L     LD    18;
      T     #Motor_current_r;
// Zähler +1
      L     #COUNTER_READ;
      INC   1;
      T     #COUNTER_READ; //Parameterwert auslesen ENDE

//Motorstrom_Max
rp44: L     #COUNTER_READ; //Parameterwert auslesen START
      L     44;
      ==I   ;
      SPBN  rp45;
      L     LW    14;
      L     W#16#1406;
      ==I   ;
      SPBN  end9;
      L     LD    18;
      T     #Motor_current_max_r;
// Zähler +1
      L     #COUNTER_READ;
      INC   1;
      T     #COUNTER_READ; //Parameterwert auslesen ENDE

//Allg_Statusregister
rp45: L     #COUNTER_READ; //Parameterwert auslesen START
      L     45;
      ==I   ;
      SPBN  rp46;
      L     LW    14;
      L     W#16#1407;
      ==I   ;
      SPBN  end9;
      L     LD    18;
      T     #Gen_Status_Register_r;
// Zähler +1
      L     #COUNTER_READ;
      INC   1;
      T     #COUNTER_READ; //Parameterwert auslesen ENDE

//Drehmoment_Abschaltung
rp46: L     #COUNTER_READ; //Parameterwert auslesen START
      L     46;
      ==I   ;
      SPBN  rp47;
      L     LW    14;
      L     W#16#1408;
      ==I   ;
      SPBN  end9;
      L     LD    18;
      T     #Torque_Deactivation_r;
// Zähler +1
      L     #COUNTER_READ;
      INC   1;
      T     #COUNTER_READ; //Parameterwert auslesen ENDE

//Seriennummer
rp47: L     #COUNTER_READ; //Parameterwert auslesen START
      L     47;
      ==I   ;
      SPBN  rp99;
      L     LW    14;
      L     W#16#2409;
      ==I   ;
      SPBN  end9;
      L     LD    18;
      T     #Serial_number_r;
// Zähler +1
      L     #COUNTER_READ;
      INC   1;
      T     #COUNTER_READ; //Parameterwert auslesen ENDE


//Zähler lesen auf null stellen
rp99: L     0;
      T     #COUNTER_READ;
      SET   ;
      R     #REFRESH;
      SPA   end9;
end9: NOP   0;



NETWORK
TITLE =read par from drv (write)

      L     #COUNTER_WRITE; //Zählerstand nach aussen geben
      T     #COUNT_WRITE; //Zählerstand nach aussen geben

//Betriebsart
      L     #COUNTER_WRITE;
      L     1;
      ==I   ;
      SPBN  pr82;
      L     LW    14;
      L     W#16#13A2;
      ==I   ;
      SPBN  pr82;
// Zähler +1
      L     #COUNTER_WRITE;
      INC   1;
      T     #COUNTER_WRITE;

//Reglerparameter_P
pr82: L     #COUNTER_WRITE;
      L     2;
      ==I   ;
      SPBN  pr83;
      L     LW    14;
      L     W#16#13E8;
      ==I   ;
      SPBN  pr83;
// Zähler +1
      L     #COUNTER_WRITE;
      INC   1;
      T     #COUNTER_WRITE;


//Reglerparameter_I
pr83: L     #COUNTER_WRITE;
      L     3;
      ==I   ;
      SPBN  pr84;
      L     LW    14;
      L     W#16#13E9;
      ==I   ;
      SPBN  pr84;
// Zähler +1
      L     #COUNTER_WRITE;
      INC   1;
      T     #COUNTER_WRITE;


//Reglerparameter_D
pr84: L     #COUNTER_WRITE;
      L     4;
      ==I   ;
      SPBN  pr85;
      L     LW    14;
      L     W#16#13EA;
      ==I   ;
      SPBN  pr85;
// Zähler +1
      L     #COUNTER_WRITE;
      INC   1;
      T     #COUNTER_WRITE;


//a_Pos
pr85: L     #COUNTER_WRITE;
      L     5;
      ==I   ;
      SPBN  pr86;
      L     LW    14;
      L     W#16#13EB;
      ==I   ;
      SPBN  pr86;
// Zähler +1
      L     #COUNTER_WRITE;
      INC   1;
      T     #COUNTER_WRITE;


//v_Pos
pr86: L     #COUNTER_WRITE;
      L     6;
      ==I   ;
      SPBN  pr87;
      L     LW    14;
      L     W#16#13EC;
      ==I   ;
      SPBN  pr87;
// Zähler +1
      L     #COUNTER_WRITE;
      INC   1;
      T     #COUNTER_WRITE;


//a_Dreh
pr87: L     #COUNTER_WRITE;
      L     7;
      ==I   ;
      SPBN  pr88;
      L     LW    14;
      L     W#16#13ED;
      ==I   ;
      SPBN  pr88;
// Zähler +1
      L     #COUNTER_WRITE;
      INC   1;
      T     #COUNTER_WRITE;


//a_Tipp
pr88: L     #COUNTER_WRITE;
      L     8;
      ==I   ;
      SPBN  pr89;
      L     LW    14;
      L     W#16#13EF;
      ==I   ;
      SPBN  pr89;
// Zähler +1
      L     #COUNTER_WRITE;
      INC   1;
      T     #COUNTER_WRITE;


//v_Tip
pr89: L     #COUNTER_WRITE;
      L     9;
      ==I   ;
      SPBN  pr90;
      L     LW    14;
      L     W#16#13F0;
      ==I   ;
      SPBN  pr90;
// Zähler +1
      L     #COUNTER_WRITE;
      INC   1;
      T     #COUNTER_WRITE;

//Pos_Fenster
pr90: L     #COUNTER_WRITE;
      L     10;
      ==I   ;
      SPBN  pr91;
      L     LW    14;
      L     W#16#13F1;
      ==I   ;
      SPBN  pr91;
// Zähler +1
      L     #COUNTER_WRITE;
      INC   1;
      T     #COUNTER_WRITE;


//ue_Zaehler
pr91: L     #COUNTER_WRITE;
      L     11;
      ==I   ;
      SPBN  pr92;
      L     LW    14;
      L     W#16#13F2;
      ==I   ;
      SPBN  pr92;
// Zähler +1
      L     #COUNTER_WRITE;
      INC   1;
      T     #COUNTER_WRITE;


//ue_Nenner
pr92: L     #COUNTER_WRITE;
      L     12;
      ==I   ;
      SPBN  pr93;
      L     LW    14;
      L     W#16#13F3;
      ==I   ;
      SPBN  pr93;
// Zähler +1
      L     #COUNTER_WRITE;
      INC   1;
      T     #COUNTER_WRITE;


//Spindelsteigung
pr93: L     #COUNTER_WRITE;
      L     13;
      ==I   ;
      SPBN  pr94;
      L     LW    14;
      L     W#16#13F4;
      ==I   ;
      SPBN  pr94;
// Zähler +1
      L     #COUNTER_WRITE;
      INC   1;
      T     #COUNTER_WRITE;


//Drehrichtung
pr94: L     #COUNTER_WRITE;
      L     14;
      ==I   ;
      SPBN  pr95;
      L     LW    14;
      L     W#16#13F5;
      ==I   ;
      SPBN  pr95;
// Zähler +1
      L     #COUNTER_WRITE;
      INC   1;
      T     #COUNTER_WRITE;


//Pos_Art_
pr95: L     #COUNTER_WRITE;
      L     15;
      ==I   ;
      SPBN  pr96;
      L     LW    14;
      L     W#16#13F6;
      ==I   ;
      SPBN  pr96;
// Zähler +1
      L     #COUNTER_WRITE;
      INC   1;
      T     #COUNTER_WRITE;


//oberer_Grenzwert
pr96: L     #COUNTER_WRITE;
      L     16;
      ==I   ;
      SPBN  pr97;
      L     LW    14;
      L     W#16#23F8;
      ==I   ;
      SPBN  pr97;
// Zähler +1
      L     #COUNTER_WRITE;
      INC   1;
      T     #COUNTER_WRITE;


//unterer_Grenzwert
pr97: L     #COUNTER_WRITE;
      L     17;
      ==I   ;
      SPBN  pr98;
      L     LW    14;
      L     W#16#23F9;
      ==I   ;
      SPBN  pr98;
// Zähler +1
      L     #COUNTER_WRITE;
      INC   1;
      T     #COUNTER_WRITE;


//Kalibrierwert
pr98: L     #COUNTER_WRITE;
      L     18;
      ==I   ;
      SPBN  pr99;
      L     LW    14;
      L     W#16#23FA;
      ==I   ;
      SPBN  pr99;
// Zähler +1
      L     #COUNTER_WRITE;
      INC   1;
      T     #COUNTER_WRITE;


//Delta_Tipp
pr99: L     #COUNTER_WRITE;
      L     19;
      ==I   ;
      SPBN  p100;
      L     LW    14;
      L     W#16#23FB;
      ==I   ;
      SPBN  p100;
// Zähler +1
      L     #COUNTER_WRITE;
      INC   1;
      T     #COUNTER_WRITE;

//Stopp-Mode Tipp2
p100: L     #COUNTER_WRITE;
      L     20;
      ==I   ;
      SPBN  p101;
      L     LW    14;
      L     W#16#13FD;
      ==I   ;
      SPBN  p101;
// Zähler +1
      L     #COUNTER_WRITE;
      INC   1;
      T     #COUNTER_WRITE;

//InPos_Mode
p101: L     #COUNTER_WRITE;
      L     21;
      ==I   ;
      SPBN  p102;
      L     LW    14;
      L     W#16#13FE;
      ==I   ;
      SPBN  p102;
// Zähler +1
      L     #COUNTER_WRITE;
      INC   1;
      T     #COUNTER_WRITE;

//Schleifenlaenge
p102: L     #COUNTER_WRITE;
      L     22;
      ==I   ;
      SPBN  p103;
      L     LW    14;
      L     W#16#13FF;
      ==I   ;
      SPBN  p103;
// Zähler +1
      L     #COUNTER_WRITE;
      INC   1;
      T     #COUNTER_WRITE;

//Schleppfehler_Grenze
p103: L     #COUNTER_WRITE;
      L     23;
      ==I   ;
      SPBN  p104;
      L     LW    14;
      L     W#16#1400;
      ==I   ;
      SPBN  p104;
// Zähler +1
      L     #COUNTER_WRITE;
      INC   1;
      T     #COUNTER_WRITE;

//Drehmoment_Abschaltung
p104: L     #COUNTER_WRITE;
      L     24;
      ==I   ;
      SPBN  p199;
      L     LW    14;
      L     W#16#1408;
      ==I   ;
      SPBN  p199;
// Zähler +1
      L     #COUNTER_WRITE;
      INC   1;
      T     #COUNTER_WRITE;

//Parametersatz laden
p199: L     #COUNTER_WRITE;
      L     25;
      ==I   ;
      SPBN  ende;
      L     W#16#23CA;
      L     LW    14;
      ==I   ;
      SPBN  ende;
//Schreiben beenden
      L     0;
      T     #COUNTER_WRITE;
      SET   ;
      S     #REFRESH;

ende: NOP   0; //ENDE


NETWORK
TITLE =ZSW 1
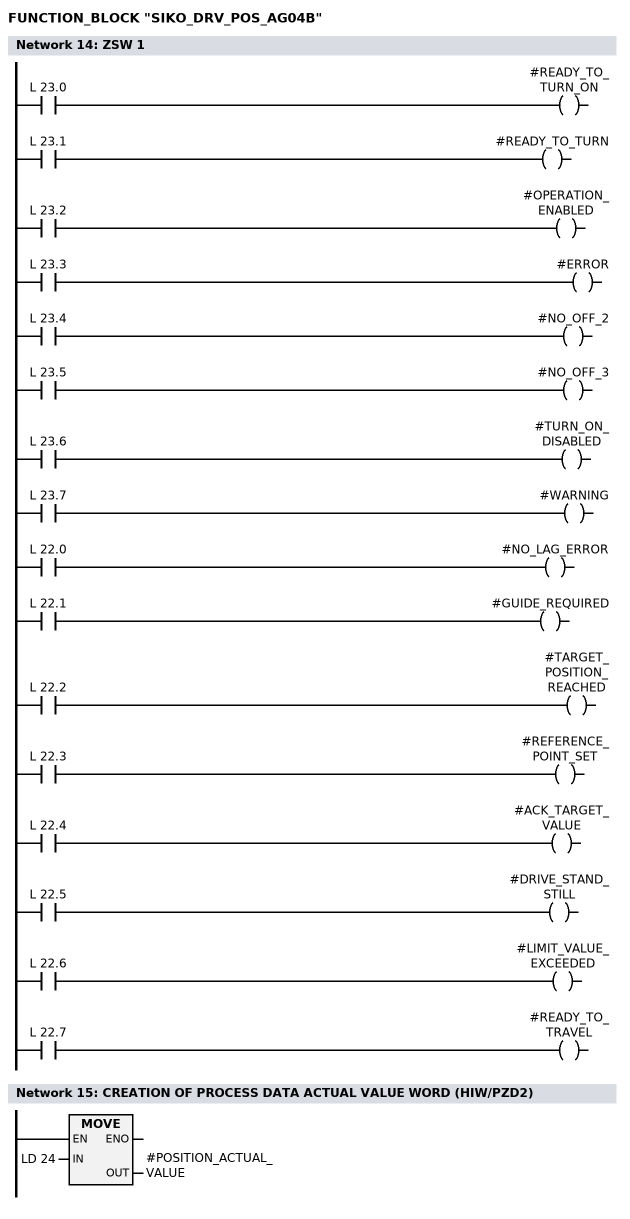
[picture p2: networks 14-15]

      U     L     23.0;
      =     #READY_TO_TURN_ON;
      U     L     23.1;
      =     #READY_TO_TURN;
      U     L     23.2;
      =     #OPERATION_ENABLED;
      U     L     23.3;
      =     #ERROR;
      U     L     23.4;
      =     #NO_OFF_2;
      U     L     23.5;
      =     #NO_OFF_3;
      U     L     23.6;
      =     #TURN_ON_DISABLED;
      U     L     23.7;
      =     #WARNING;
      U     L     22.0;
      =     #NO_LAG_ERROR;
      U     L     22.1;
      =     #GUIDE_REQUIRED;
      U     L     22.2;
      =     #TARGET_POSITION_REACHED;
      U     L     22.3;
      =     #REFERENCE_POINT_SET;
      U     L     22.4;
      =     #ACK_TARGET_VALUE;
      U     L     22.5;
      =     #DRIVE_STAND_STILL;
      U     L     22.6;
      =     #LIMIT_VALUE_EXCEEDED;
      U     L     22.7;
      =     #READY_TO_TRAVEL;


NETWORK
TITLE =CREATION OF PROCESS DATA ACTUAL VALUE WORD (HIW/PZD2)
//
      L     LD    24;
      T     #POSITION_ACTUAL_VALUE;

END_FUNCTION_BLOCK

